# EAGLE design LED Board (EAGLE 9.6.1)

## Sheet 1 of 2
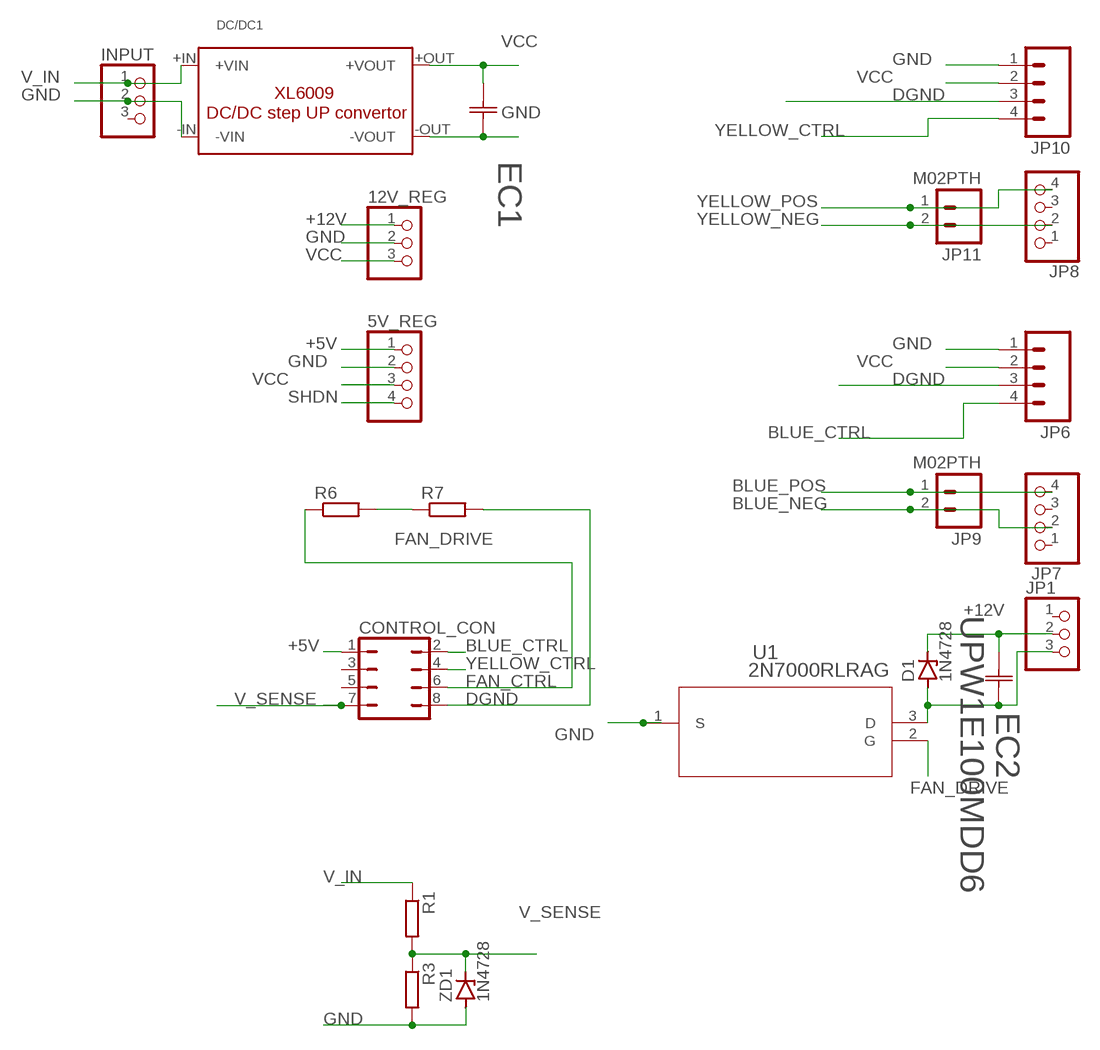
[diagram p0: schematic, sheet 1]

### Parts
5V_REG  PINHD-1X4  [1X04]
12V_REG  PINHD-1X3  [1X03]
CONTROL_CON  JP4Q  [JP4Q]
D1  1N4728  [DO41Z10]
DC/DC1  DC/DC-STEP-UP-XL6009  [DC/DC-STEP-UP-XL6009]
EC1  50YXJ100MT78X11.5  [CAP_YX_8X11P5_RUB]
EC2  UPW1E100MDD6  [U1-A_NCH]
INPUT  PINHD-1X3  [1X03]
JP1  PINHD-1X3  [1X03]
JP6  M04PTH  [1X04]
JP7  PINHD-1X4  [1X04]
JP8  PINHD-1X4  [1X04]
JP9  M02PTH  [1X02]
JP10  M04PTH  [1X04]
JP11  M02PTH  [1X02]
R1  R-EU_0207/7  [0207/7]
R3  R-EU_0207/7  [0207/7]
R6  R-EU_0207/7  [0207/7]
R7  R-EU_0207/7  [0207/7]
U1  2N7000RLRAG  [TO-92_ONS]
ZD1  1N4728  [DO41Z10]

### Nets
+5V [Low Power]: 5V_REG.1 CONTROL_CON.1
+12V [Low Power]: 12V_REG.1 D1.C EC2.1 JP1.2
BLUE_CTRL: CONTROL_CON.2 JP6.4
BLUE_NEG: JP7.2 JP9.2
BLUE_POS: JP7.4 JP9.1
DGND: CONTROL_CON.8 JP6.3 JP10.3 R7.2
FAN_CTRL: CONTROL_CON.6 R6.1
FAN_DRIVE: R6.2 R7.1 U1.2(G)
GND [Low Power]: 5V_REG.2 12V_REG.2 DC/DC1.-IN(-VIN) DC/DC1.-OUT(-VOUT) EC1.2 INPUT.2 JP6.1 JP10.1 R3.2 U1.1(S) ZD1.A
N$2: D1.A EC2.2 JP1.3 U1.3(D)
SHDN [High Power]: 5V_REG.4
V_IN: DC/DC1.+IN(+VIN) INPUT.1 R1.1
V_SENSE: CONTROL_CON.7 R1.2 R3.1 ZD1.C
VCC [High Power]: 5V_REG.3 12V_REG.3 DC/DC1.+OUT(+VOUT) EC1.1 JP6.2 JP10.2
YELLOW_CTRL: CONTROL_CON.4 JP10.4
YELLOW_NEG: JP8.2 JP11.2
YELLOW_POS: JP8.4 JP11.1
Unconnected: CONTROL_CON.3 CONTROL_CON.5 INPUT.3 JP1.1 JP7.1 JP7.3 JP8.1 JP8.3

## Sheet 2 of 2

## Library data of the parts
5V_REG JP7 JP8 = pinhead:PINHD-1X4: PIN HEADER
12V_REG JP1 = Silent_Headers:PINHD-1X3: PIN HEADER
CONTROL_CON = Jumper_Silent:JP4Q: JUMPER
D1 ZD1 = diode:1N4728: Z DIODE
DC/DC1 = hacesoft:DC/DC-STEP-UP-XL6009
EC1 = Added Capacitors:50YXJ100MT78X11.5: CAP ALUM 100UF 20% 50V RADIAL; BUILT_BY: EMA_Cory; COPYRIGHT: Copyright (C) 2018 Accelerated Designs. All rights reserved; MANUFACTURER_PART_NUMBER: 50YXJ100MT78X11.5; SOURCELIBRARY: Rubycon_2019-09-19; VENDOR: Rubycon Netherlands
EC2 = Digikey Components:UPW1E100MDD6: UPW1E100MDD6 10uF 25V Electrolytic Capacitor; BUILT_BY: EMA_UL_Team; MANUFACTURER_PART_NUMBER: UPW1E100MDD6; SOURCELIBRARY: Nichicon_2014-12-31; VENDOR: Nichicon
INPUT = pinhead:PINHD-1X3: PIN HEADER
JP6 JP10 = SparkFun-Connectors:M04: Header 4 Standard 4-pin 0.1" header. Use with straight break away headers (SKU : PRT-00116), right angle break away headers (PRT-00553), swiss pins (PRT-00743), machine pins (PRT-00117), and female headers (PRT-00115). Molex polarized connector foot print use with SKU : PRT-08231 with associated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
JP9 JP11 = SparkFun-Connectors:M02: Standard 2-pin 0.1" header. Use with
R1 R3 R6 R7 = rcl:R-EU_: RESISTOR, European symbol; SPICEPREFIX: R
U1 = Digikey Components:2N7000RLRAG: 2N7000 N-Channel MOSFET; BUILT_BY: EMA_UL_Team; MANUFACTURER_PART_NUMBER: 2N7000RLRAG; SOURCELIBRARY: ON_Semi_2010-01-01; VENDOR: ON Semiconductor

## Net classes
0 default: width 0.254 mm
1 High Power: width 1.27 mm
2 Low Power: width 0.254 mm

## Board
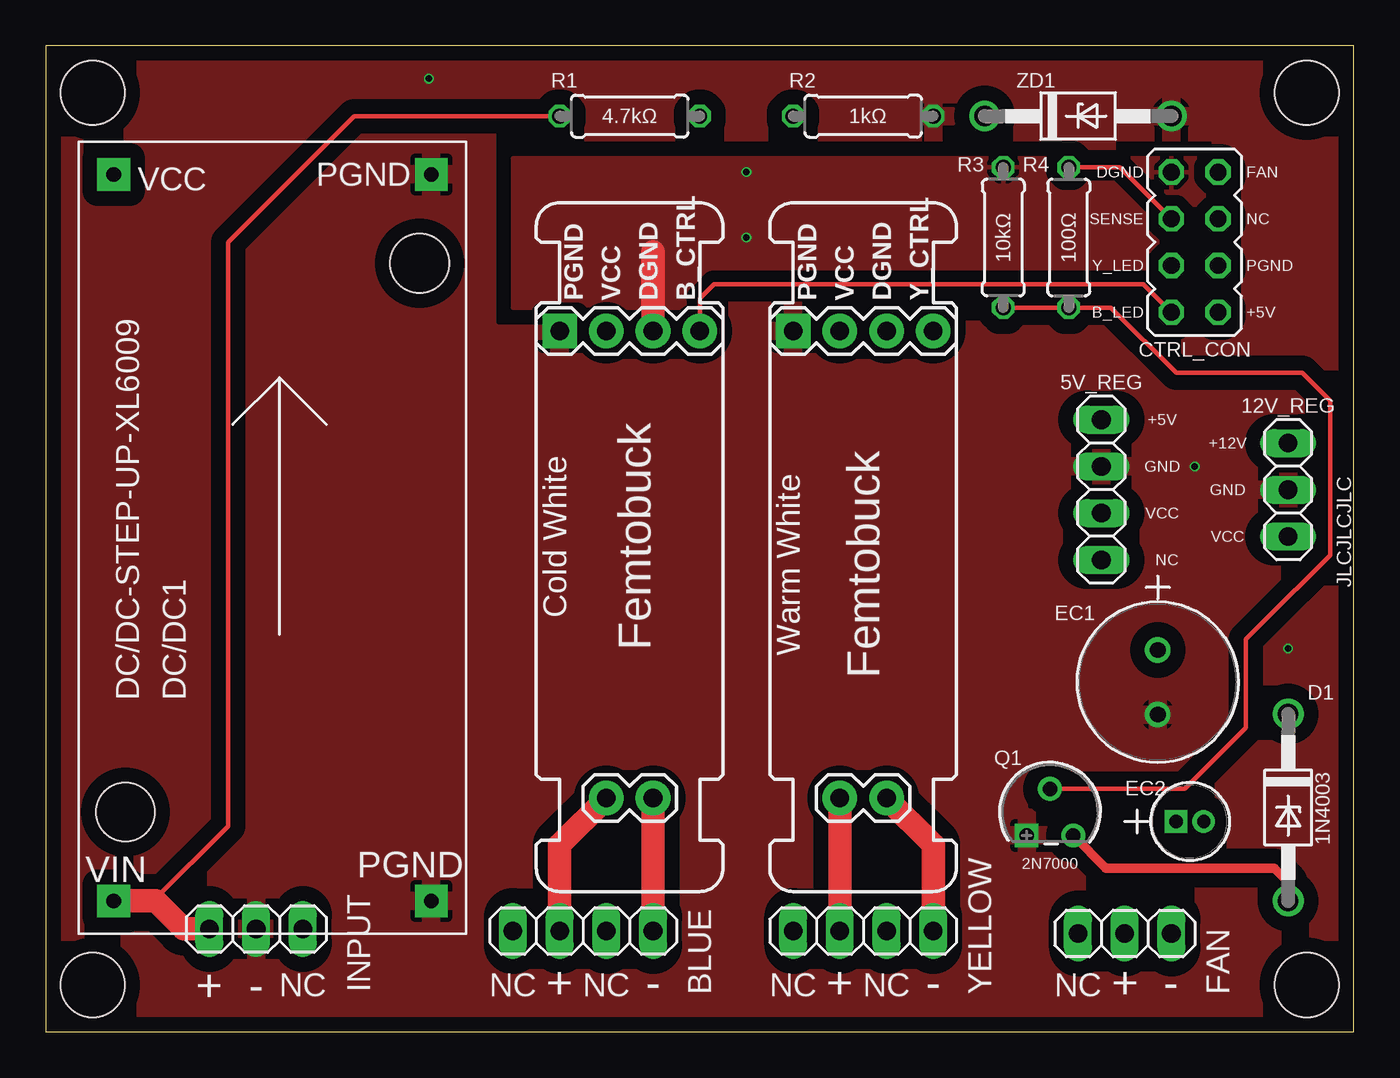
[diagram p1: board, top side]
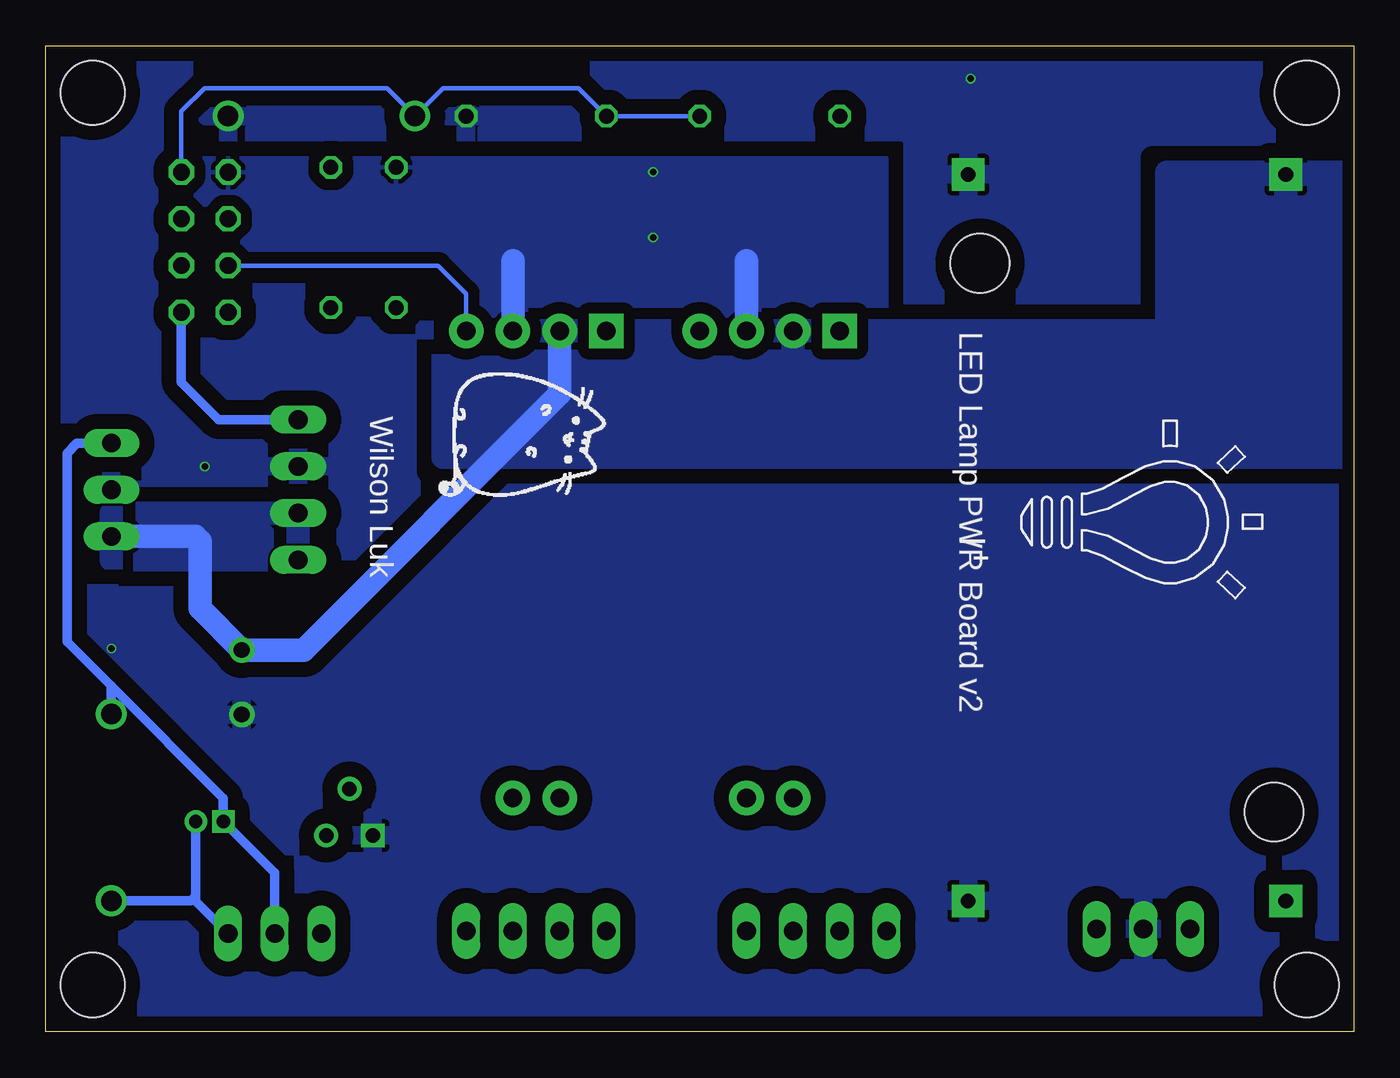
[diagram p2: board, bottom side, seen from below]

Size 71.12 x 53.59 mm. Coordinates in mm from the lower left corner, seen from the top.
Outline: 0,0 71.12,0 71.12,53.59 0,53.59 0,0
Copper layers (1*16): Top 0.035559375mm / dielectric 1.6mm / Bottom 0.035559375mm
Design rules "jlcpcb2layer": minimum track width 5mil, minimum drill 12mil, track to track 5mil, track to pad 5mil, pad to pad 5mil, via to via 5mil, smd to smd 5mil, copper to edge 8mil, drill to drill 6mil, minimum pad ring 5mil, minimum via ring 3mil, stop-mask expansion 2.5mil, vias tented up to drill 0mil, thermal gap 10mil
Holes 3.5 mm at 68.58,2.54 68.58,51.05 2.54,51.05 2.54,2.54

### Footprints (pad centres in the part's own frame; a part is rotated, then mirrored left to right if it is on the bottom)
1X04 = drill 1.016 long: 1 -3.81,0; 2 -1.27,0; 3 1.27,0; 4 3.81,0
1X03 = drill 1.016 long: 1 -2.54,0; 2 0,0; 3 2.54,0
JP4Q = drill 0.914 octagon: 1 -3.81,-1.27; 2 -3.81,1.27; 3 -1.27,-1.27; 4 -1.27,1.27; 5 1.27,-1.27; 6 1.27,1.27; 7 3.81,-1.27; 8 3.81,1.27
DO41Z10 = drill 1.118: A 5.08,0; C -5.08,0
DC/DC-STEP-UP-XL6009 = drill 0.8 pad 1.778 square: +IN 1.778,19.177; +OUT 41.275,19.177; -IN 1.778,1.905; -OUT 41.275,1.905 | hole 3.2: 6.604,18.542; 36.449,2.54
CAP_YX_8X11P5_RUB = drill 0.864 pad 1.372: 1 0,0; 2 3.505,0
U1-A_NCH = drill 0.711 pad 1.219 square: 1 0,0 | drill 0.711 pad 1.219: 2 1.499,0
1X04' = drill 1.016 pad 1.88 square: 1 0,0 | drill 1.016 pad 1.88: 2 2.54,0; 3 5.08,0; 4 7.62,0
1X02 = drill 1.016 pad 1.88: 1 0,0; 2 2.54,0
0207/7 = drill 0.813 octagon: 1 -3.81,0; 2 3.81,0
TO-92_ONS = drill 0.787 pad 1.295 square: 1 0,0 | drill 0.787 pad 1.295: 2 1.27,2.54; 3 2.54,0

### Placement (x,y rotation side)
5V_REG  57.4,29.46 270 top
12V_REG  67.56,29.46 270 top
CONTROL_CON  62.48,42.93 90 top
D1  67.56,12.19 270 top
DC/DC1  22.86,5.33 90 top
EC1  60.47,20.75 270 top
EC2  61.47,11.43 0 top
INPUT  11.43,5.59 0 top
JP1  58.67,5.33 0 top
JP6  [1X04']  27.94,38.1 0 top
JP7  29.21,5.48 0 top
JP8  44.45,5.48 0 top
JP9  33.02,12.7 180 top
JP10  [1X04']  40.64,38.1 0 top
JP11  45.72,12.7 180 top
R1  31.75,49.78 0 top
R3  44.45,49.78 0 top
R6  55.63,43.18 270 top
R7  52.07,43.18 90 top
U1  53.34,10.67 0 top
ZD1  56.13,49.78 0 top

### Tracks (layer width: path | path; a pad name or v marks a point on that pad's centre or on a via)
+5V
  Bottom 0.508: 5V_REG.1 61.72,33.27 63.75,35.31 CONTROL_CON.1
+12V
  Bottom 0.508: 12V_REG.1 69.43,32 69.98,31.46 69.98,21.21 67.56,18.8 | 67.56,18.8 D1.C 67.56,18.8 | 67.56,18.8 61.47,12.7 EC2.1 58.67,8.64 JP1.2
BLUE_CTRL
  Top 0.254: CONTROL_CON.2 59.69,40.64 36.32,40.64 35.56,39.88 JP6.4
BLUE_NEG
  Top 1.27: JP7.2 27.94,10.16 JP9.2
BLUE_POS
  Top 1.27: JP9.1 JP7.4
DGND  (via drill 0.35)
  Top 1.27: JP6.3 33.02,42.42
  Bottom 1.27: 45.72,41.91 JP10.3 | 33.02,41.91 JP6.3
  other vias: 38.1,43.18 38.1,46.74
  pour Bottom (isolate 0.61, rank 2): 25.4,47.5 25.4,38.61 51.05,38.61 51.05,37.08 65.02,37.08 65.02,47.5
  pour Top (isolate 0.61): 25.4,47.5 25.4,39.37 51.05,39.37 51.05,37.08 65.02,37.08 65.02,47.5
FAN_CTRL
  Top 0.254: CONTROL_CON.6 58.42,46.99 R6.1
FAN_DRIVE
  Top 0.254: R7.1 R6.2 57.91,39.37 61.47,35.81 68.34,35.81 69.85,34.31 69.85,25.91 66.12,22.17 66.1,22.17 65.27,21.35 65.27,16.52 61.95,13.21 U1.2
GND  (via drill 0.35)
  other vias: 62.48,30.73 20.83,51.82 67.56,20.83
  pour Bottom (isolate 0.813, rank 3): 0,53.59 0,0 71.12,0 71.12,53.59
  pour Top (isolate 0.813, rank 2): 0,53.59 0,0 71.12,0 71.12,53.59
N$2
  Top 0.508: D1.A 67.56,8.13 66.8,8.89 57.66,8.89 U1.3
  Bottom 0.508: JP1.3 62.97,7.09 EC2.2 62.97,7.39 63.25,7.11 D1.A
V_IN
  Top 0.254: R1.1 16.76,49.78 9.91,42.93 9.91,11.18 5.84,7.11 DC/DC1.+IN
  Top 1.27: DC/DC1.+IN 5.97,7.11 7.49,5.59 INPUT.1
V_SENSE
  Bottom 0.254: R1.2 R3.1 42.16,51.31 49.53,51.31 ZD1.C 52.58,51.31 62.48,51.31 63.75,50.04 CONTROL_CON.7
VCC
  Bottom 0.508: EC1.1 60.39,20.83
  Bottom 1.27: 65.37,26.92 12V_REG.3 62.99,26.92 62.74,26.67 62.74,23.02 EC1.1 57.1,20.75 43.18,34.67 JP10.2
  pour Bottom (isolate 0.61): 0,46.72 10.16,46.72 10.16,38.35 10.41,38.1 49.53,38.1 49.53,31.24 -0.02,31.24
  pour Bottom: 57.4,28.19 57.4,25.65 67.56,25.65 67.56,28.19
YELLOW_CTRL
  Bottom 0.254: JP10.4 48.26,40.13 49.78,41.66 CONTROL_CON.4
YELLOW_NEG
  Top 1.27: JP8.2 JP11.2
YELLOW_POS
  Top 1.27: JP11.1 48.26,10.16 JP8.4

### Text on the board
tPlace: R1 | R2 | ZD1 | 4.7kΩ | 1kΩ | R3 | R4 | DGND | FAN | VCC | PGND | SENSE | NC | 10kΩ | 100Ω | Y_LED | PGND | PGND | VCC | DGND | B_CTRL | PGND | VCC | DGND | Y_CTRL | B_LED | +5V | CTRL_CON | 5V_REG | 12V_REG | +5V | +12V | GND | GND | VCC | Cold White | Femtobuck | VCC | JLCJLCJLC | NC | Warm White | Femtobuck | EC1 | D1 | Q1 | 1N4003 | 2N7000 | VIN | PGND | + | - | NC | NC | + | NC | - | NC | + | NC | - | NC | + | - | BLUE | YELLOW | FAN
bPlace: Wilson Luk | LED Lamp PWR Board v2
Measures: (typ.) | (typ.) | Units are inches | Units are inches

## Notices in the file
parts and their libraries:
SparkFun-Connectors: Licensing: Creative Commons ShareAlike 4.0 International - https://creativecommons.org/licenses/by-sa/4.0
